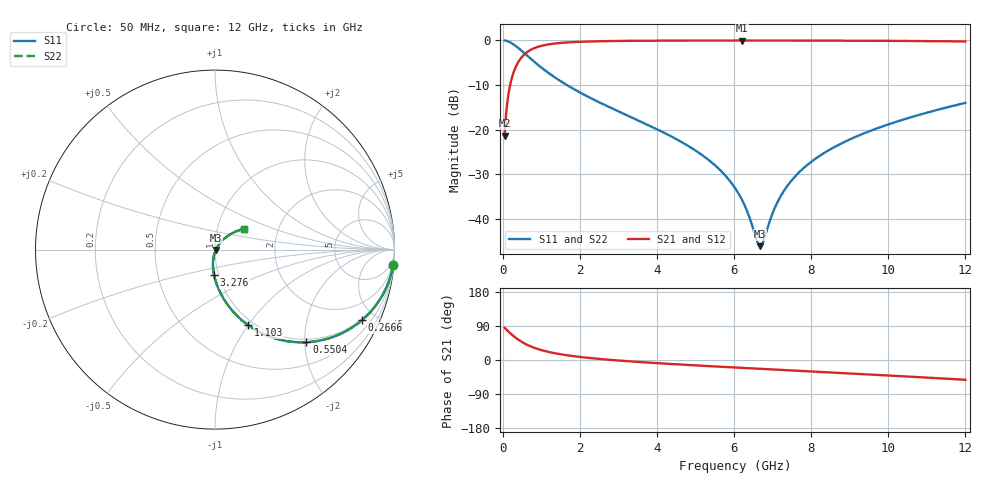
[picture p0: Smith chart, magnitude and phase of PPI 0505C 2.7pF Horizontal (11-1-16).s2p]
# MHz S MA R 50
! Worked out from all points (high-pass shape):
!   1601 points, 50 MHz to 12 GHz, reference 50 ohm
!   highest |S21| = -0.05 dB at 6.197 GHz (marker M1); lowest = -21.4 dB at 50 MHz (marker M2)
!   |S21| within 3 dB of the highest: 576.4 MHz to end of sweep
!   lowest |S11| = -46.1 dB at 6.682 GHz (marker M3), VSWR 1.01, Z = 50.5 - j0.195 ohm
!   |S11| at or under -10 dB: 1.663 GHz to end of sweep
!   |S22| runs from -46.1 to 0.0 dB; largest |S21 - S12| = 0
!   S11 on the Smith chart (normalised r, x): 50 MHz: 1, -23; 266.6 MHz: 0.93, -4.22; 550.4 MHz: 0.94, -2.03; 1.103 GHz: 0.94, -1.00; 3.276 GHz: 0.95, -0.27; 12 GHz: 1.34, +0.32
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50  0.9963 -5.1  0.08541 84.9  0.08541 84.9  0.9963 -5.1
162.0312  0.9634 -16.1  0.2677 73.9  0.2677 73.9  0.9634 -16.1
266.5938  0.9091 -25.5  0.416 64.4  0.416 64.4  0.9091 -25.5
550.4062  0.7249 -45.4  0.6876 44.5  0.6876 44.5  0.7249 -45.4
804.3438  0.5821 -57.1  0.8115 32.7  0.8115 32.7  0.5821 -57.1
1103.094  0.4591 -66.3  0.8864 23.4  0.8864 23.4  0.4591 -66.3
2044.156  0.2553 -81.8  0.9641 7.6  0.9641 7.6  0.2553 -81.8
3276.5  0.1415 -92.1  0.9864 -3.4  0.9864 -3.4  0.1415 -92.1
4038.312  0.09937 -96.4  0.9911 -8.5  0.9911 -8.5  0.09937 -96.4
5270.656  0.04836 -100.6  0.9942 -15.7  0.9942 -15.7  0.04836 -100.6
6025  0.02224 -97.8  0.9947 -19.8  0.9947 -19.8  0.02224 -97.8
6196.781  0.01667 -94.2  0.9947 -20.7  0.9947 -20.7  0.01667 -94.2
6600.094  0.005593 -51.2  0.9947 -22.9  0.9947 -22.9  0.005593 -51.2
6682.25  0.004965 -22.8  0.9946 -23.3  0.9946 -23.3  0.004965 -22.8
6764.406  0.005698 4.8  0.9946 -23.7  0.9946 -23.7  0.005698 4.8
7048.219  0.01303 41.5  0.9943 -25.2  0.9943 -25.2  0.01303 41.5
7257.344  0.01951 48.1  0.9941 -26.3  0.9941 -26.3  0.01951 48.1
7585.969  0.03002 51.6  0.9937 -28.0  0.9937 -28.0  0.03002 51.6
8019.156  0.04419 52.4  0.9929 -30.3  0.9929 -30.3  0.04419 52.4
8863.125  0.07286 50.4  0.9907 -34.7  0.9907 -34.7  0.07286 50.4
10013.31  0.115 45.7  0.986 -40.9  0.986 -40.9  0.115 45.7
12000  0.1995 35.5  0.971 -52.2  0.971 -52.2  0.1995 35.5
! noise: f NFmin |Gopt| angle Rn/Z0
50  0.0007394  0.9382  1.811  0.002668
1372  0.005708  0.7614  5.742  0.00484
2701  0.009215  0.7167  10.15  0.006381
4031  0.01235  0.6909  14.59  0.007654
5360  0.01533  0.6744  18.99  0.008835
6682  0.01824  0.6642  23.3  0.01
8012  0.02121  0.6586  27.54  0.01122
9341  0.02427  0.657  31.68  0.01253
1.067e+04  0.02748  0.6587  35.72  0.01399
1.2e+04  0.03092  0.6633  39.65  0.01565
